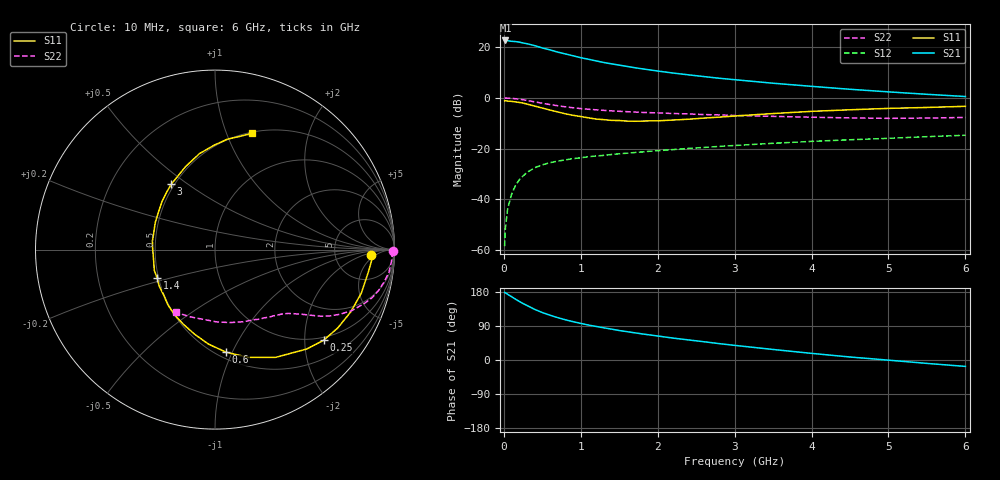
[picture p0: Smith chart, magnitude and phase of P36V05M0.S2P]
! SIEMENS Small Signal Semiconductors
! BFP181
! Si NPN RF Bipolar Junction Transistor in SOT143
! VCE = 6 V  IC = 5 mA
! Common Emitter S-Parameters:  March  1996
# GHz  S  MA  R  50
!  f  S11  S21  S12  S22
! GHz  MAG  ANG  MAG  ANG  MAG  ANG  MAG  ANG
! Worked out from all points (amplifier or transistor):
!   36 points, 10 MHz to 6 GHz, reference 50 ohm
!   highest |S21| = 22.6 dB at 20 MHz (marker M1)
!   |S21| within 3 dB of that: start of sweep to 506.6 MHz
!   unconditionally stable (mu >= 1): 1.782 GHz to end of sweep
!   at 250 MHz: K = 0.20, MSG = 26.2 dB, |S12| = -30.8 dB
!   at 1.4 GHz: K = 0.88, MSG = 17.8 dB, |S12| = -22.3 dB
!   at 6 GHz: K = 1.05, MAG = 6.2 dB, |S12| = -14.7 dB
!   lowest NFmin = 1.55 dB at 450 MHz
!   S11 on the Smith chart (normalised r, x): 10 MHz: 13, -3; 250 MHz: 0.92, -2.46; 600 MHz: 0.55, -0.95; 1.4 GHz: 0.49, -0.18; 3 GHz: 0.48, +0.43; 6 GHz: 0.51, +1.24
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0.01  0.8685 -1.9  13.34 178.2  0.0012 88.9  0.9908 -0.6
0.02  0.8765 -3.4  13.47 177.4  0.0027 85.2  0.9888 -1.4
0.05  0.8638 -8.2  13.36 173.3  0.0066 89.8  0.9856 -3.7
0.15  0.8322 -24.6  12.83 160.7  0.0186 75.5  0.9598 -10.8
0.2  0.8116 -32.5  12.51 154.7  0.0242 72.1  0.9398 -14.0
0.25  0.7885 -39.8  12.01 148.9  0.0289 69.1  0.9153 -17.0
0.3  0.7537 -47.3  11.63 144.0  0.034 65.5  0.8887 -19.5
0.4  0.6887 -60.7  10.67 133.6  0.0419 59.3  0.8338 -24.1
0.5  0.6286 -72.8  9.595 125.3  0.048 54.7  0.7816 -27.5
0.6  0.5751 -83.8  8.789 118.1  0.0528 51.4  0.7373 -30.1
0.7  0.5276 -94.0  7.944 111.8  0.0568 48.4  0.698 -32.1
0.8  0.4844 -103.7  7.322 106.1  0.06 46.2  0.6647 -33.6
0.9  0.4524 -112.8  6.724 101.1  0.0636 44.6  0.6368 -34.9
1.1  0.4038 -130.7  5.749 92.2  0.0694 42.3  0.5957 -37.1
1.4  0.3594 -153.9  4.669 81.5  0.0766 40.1  0.5538 -40.1
1.8  0.3482 177.6  3.724 68.8  0.086 38.8  0.5163 -44.1
2.2  0.3654 155.6  3.075 57.8  0.0956 37.0  0.4911 -48.8
3  0.438 123.9  2.276 38.6  0.1152 33.2  0.4492 -60.2
3.5  0.4904 109.6  1.939 27.8  0.1273 30.5  0.4316 -68.7
4.5  0.5817 90.5  1.473 7.9  0.1493 24.0  0.4027 -89.0
5.5  0.6464 77.5  1.173 -9.0  0.1718 18.4  0.3996 -110.6
6  0.6803 72.3  1.061 -16.9  0.1834 14.8  0.4112 -121.8
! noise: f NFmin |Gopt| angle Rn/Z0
0.45  1.55  0.48  17  0.36
0.9  1.65  0.4  35  0.34
1.8  2  0.18  88  0.34
